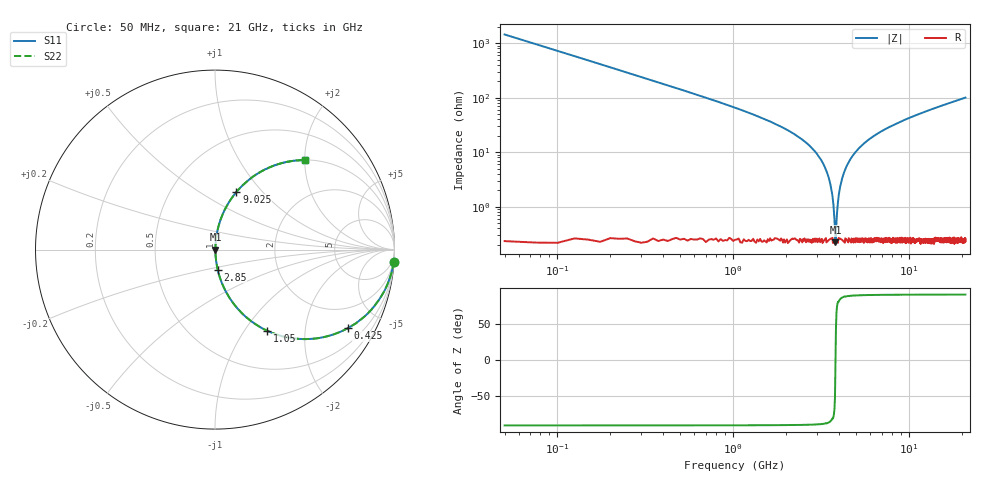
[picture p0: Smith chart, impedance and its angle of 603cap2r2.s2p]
! AVX Thin Film Operation		Date: November 2004
! Description: Accu-P® Series, Thin Film, SMD, RF Capacitor
! Part Number: 06035J2R2ABT
! 50 MHz  -  10.05 GHz
! Serial Measurements
# MHZ S MA R 50
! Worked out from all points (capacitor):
!   839 points, 50 MHz to 21 GHz, reference 50 ohm
!   read as one part in series: C = 2.2 pF near 150 MHz
!   lowest |Z| = 222 mohm at 3.825 GHz (marker M1)
!   series resonance near 3.828 GHz, so ESL is about 790 pH
!   S11 on the Smith chart (normalised r, x): 50 MHz: 1, -29; 425 MHz: 1.00, -3.36; 1.05 GHz: 1.01, -1.27; 2.85 GHz: 1.00, -0.23; 9.025 GHz: 1.00, +0.73; 21 GHz: 1.01, +2.00
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50  0.998 -4.0  0.069 86.0  0.069 86.0  0.998 -4.0
225  0.954 -17.3  0.298 72.6  0.298 72.6  0.954 -17.3
425  0.859 -30.7  0.511 59.2  0.511 59.2  0.859 -30.7
1050  0.536 -57.3  0.842 32.4  0.842 32.4  0.536 -57.3
1750  0.31 -71.5  0.948 18.1  0.948 18.1  0.31 -71.5
2850  0.112 -82.3  0.991 6.4  0.991 6.4  0.112 -82.3
3275  0.059 -84.3  0.996 3.4  0.996 3.4  0.059 -84.3
3550  0.029 -83.5  0.997 1.6  0.997 1.6  0.029 -83.5
3650  0.018 -81.4  0.997 1.0  0.997 1.0  0.018 -81.4
3750  0.008102 -72.3  0.998 0.4  0.998 0.4  0.008102 -72.3
3825  0.002414 -6.4  0.998 0.0  0.998 0.0  0.002414 -6.4
3900  0.007449 70.8  0.998 -0.4  0.998 -0.4  0.007449 70.8
4000  0.017 80.8  0.997 -1.0  0.997 -1.0  0.017 80.8
4150  0.031 83.8  0.997 -1.7  0.997 -1.7  0.031 83.8
4650  0.074 83.9  0.995 -4.2  0.995 -4.2  0.074 83.9
5575  0.144 80.8  0.987 -8.3  0.987 -8.3  0.144 80.8
7050  0.238 75.7  0.969 -13.8  0.969 -13.8  0.238 75.7
9025  0.343 69.6  0.937 -20.0  0.937 -20.0  0.343 69.6
10525  0.41 65.5  0.91 -24.2  0.91 -24.2  0.41 65.5
14025  0.539 57.2  0.84 -32.6  0.84 -32.6  0.539 57.2
17525  0.635 50.4  0.771 -39.4  0.771 -39.4  0.635 50.4
21000  0.707 44.9  0.705 -45.0  0.705 -45.0  0.707 44.9
